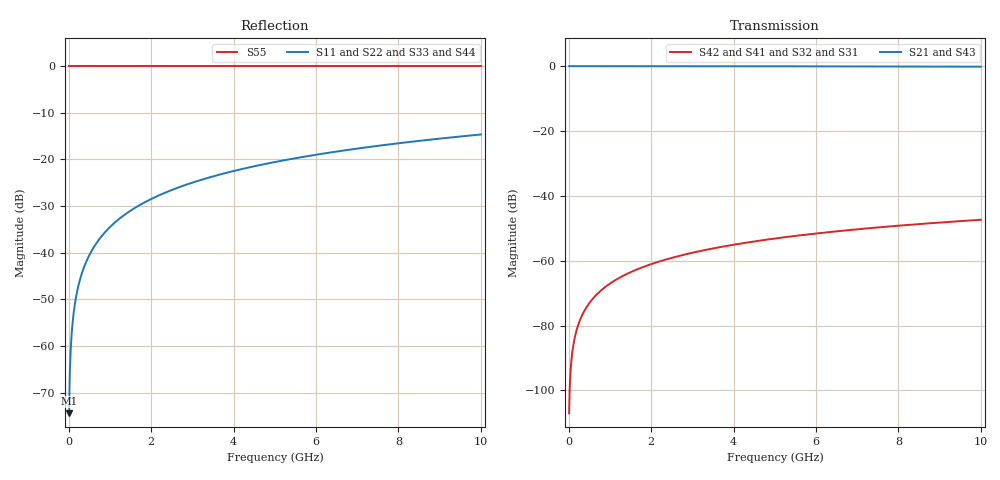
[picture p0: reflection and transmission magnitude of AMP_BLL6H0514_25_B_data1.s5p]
! Created Wed Apr 14 10:37:46 2010
# ghz S ma R 50
! 5 Port Network Data from SP1.SP block
! freq  magS11  angS11  magS12  angS12  magS13  angS13  magS14  angS14
!  magS15  angS15
!  magS21  angS21  magS22  angS22  magS23  angS23
!  magS24  angS24  magS25  angS25
!  magS31  angS31  magS32  angS32
!  magS33  angS33  magS34  angS34  magS35  angS35
!  magS41  angS41
!  magS42  angS42  magS43  angS43  magS44  angS44  magS45  angS45
!  magS51  angS51  magS52  angS52  magS53  angS53  magS54  angS54
!  magS55  angS55
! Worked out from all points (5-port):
!   1000 points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, 10 MHz to 10 GHz, reference 50 ohm
!   strongest paths, dB at 10 MHz, 2.51 GHz, 5.01 GHz, 7.51 GHz, 10 GHz:
!     S21: 0.0, 0.0, 0.0, -0.1, -0.2
!     S43: 0.0, 0.0, 0.0, -0.1, -0.2
!     S42: -107.0, -59.1, -53.1, -49.7, -47.4
!     S41: -107.0, -59.1, -53.1, -49.7, -47.4
!     S32: -107.0, -59.1, -53.1, -49.7, -47.4
!     S31: -107.0, -59.1, -53.1, -49.7, -47.4
!   lowest |S11| = -74.4 dB at 10 MHz (marker M1), VSWR 1.00, Z = 50 + j0.0189 ohm
!   |S11| at or under -10 dB: start of sweep to end of sweep
